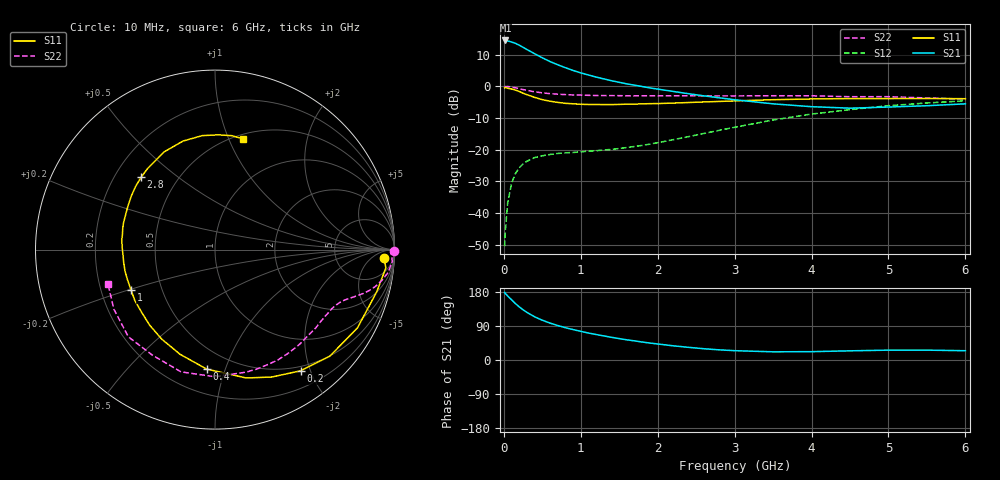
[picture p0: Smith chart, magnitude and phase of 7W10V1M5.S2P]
! Infineon Technologies  Discrete & RF Semiconductors
! BFS17W
! Si NPN RF Bipolar Junction Transistor in SOT323
! VCE = 10 V  IC = 1.5 mA
! Common Emitter S-Parameters:  August  1999
# GHz  S  MA  R  50
!  f  S11  S21  S12  S22
! GHz  MAG  ANG  MAG  ANG  MAG  ANG  MAG  ANG
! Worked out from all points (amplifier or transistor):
!   36 points, 10 MHz to 6 GHz, reference 50 ohm
!   highest |S21| = 14.4 dB at 20 MHz (marker M1)
!   |S21| within 3 dB of that: start of sweep to 311.7 MHz
!   unconditionally stable (mu >= 1): 952 MHz to 2.782 GHz; 4.313 GHz to end of sweep
!   at 250 MHz: K = 0.30, MSG = 18.4 dB, |S12| = -24.5 dB
!   at 1.4 GHz: K = 1.25, MAG = 7.8 dB, |S12| = -19.9 dB
!   at 6 GHz: K = 1.08, MAG = -2.2 dB, |S12| = -4.6 dB
!   S11 on the Smith chart (normalised r, x): 10 MHz: 20, -17; 200 MHz: 0.43, -1.85; 400 MHz: 0.36, -0.87; 1 GHz: 0.33, -0.20; 2.8 GHz: 0.31, +0.37; 6 GHz: 0.54, +1.13
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0.01  0.9432 -2.9  5.246 178.4  0.003 81.8  0.9999 -0.3
0.02  0.9574 -6.1  5.278 175.6  0.0053 89.1  0.9828 -1.4
0.05  0.9311 -14.7  5.191 169.0  0.0145 81.9  0.9902 -3.9
0.1  0.9057 -28.8  4.991 159.0  0.0292 74.4  0.9732 -7.5
0.15  0.8726 -42.9  4.761 148.9  0.0418 66.9  0.9454 -10.5
0.2  0.8265 -54.8  4.447 140.3  0.0519 61.9  0.9163 -13.0
0.25  0.7775 -65.9  4.117 132.5  0.0596 55.8  0.8868 -15.0
0.3  0.7363 -76.3  3.805 125.7  0.0656 52.3  0.8609 -16.5
0.4  0.6673 -94.0  3.259 114.0  0.0749 46.1  0.8171 -18.8
0.5  0.615 -108.4  2.814 105.0  0.0801 42.9  0.7867 -20.5
0.6  0.5807 -120.6  2.454 97.4  0.0838 41.0  0.7647 -22.0
0.7  0.5568 -130.8  2.183 91.0  0.087 40.6  0.7504 -23.5
0.8  0.5376 -139.6  1.964 85.3  0.089 40.3  0.738 -25.2
1  0.5192 -154.3  1.625 75.7  0.0926 42.0  0.7254 -28.4
1.1  0.5158 -161.1  1.505 71.1  0.0945 43.6  0.7188 -30.5
1.6  0.522 174.3  1.09 53.2  0.1079 54.0  0.7068 -40.9
2.2  0.5426 153.4  0.829 37.5  0.1433 66.5  0.707 -55.2
2.8  0.5761 135.6  0.657 26.8  0.2017 71.6  0.7052 -70.9
3.5  0.6138 117.5  0.528 21.6  0.2935 69.7  0.7087 -89.9
4.5  0.639 96.4  0.451 24.2  0.4273 57.9  0.6838 -120.6
5.5  0.6416 81.5  0.493 26.0  0.5445 44.0  0.654 -149.4
6  0.6361 75.8  0.528 24.5  0.5901 37.2  0.6264 -162.4
